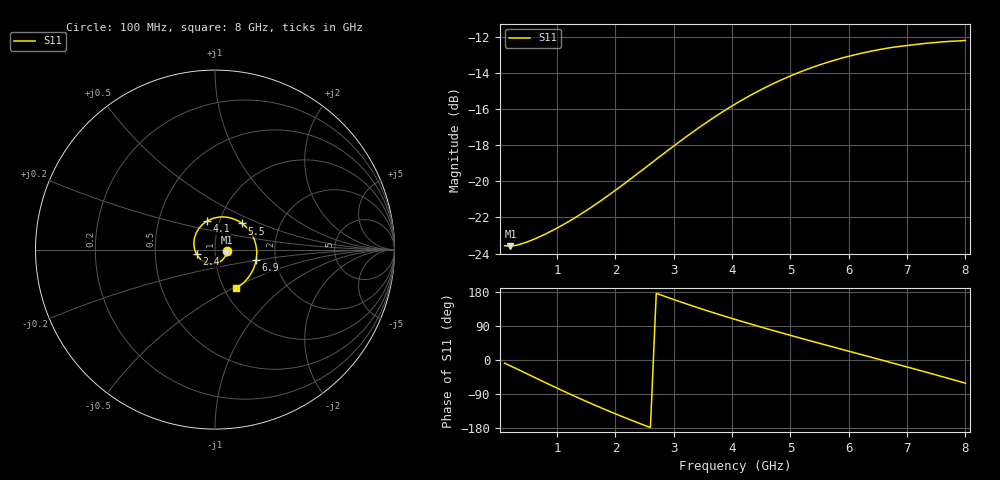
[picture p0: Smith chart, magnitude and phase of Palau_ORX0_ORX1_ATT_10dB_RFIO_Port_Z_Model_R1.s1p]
! Created Fri Oct  9 14:28:06 2020
! Palau ORX0/ORX1 RFIO Port Impedance Model.
! Attenuation  : 10 dB.
! Revision		: R1.
! Impedance Mode 	: Balanced Differential-Mode.
! Impedance Format 	: Series Equivalent Differential Impedance (SEDZ).
# hz S ma R 100
! 1 Port Network Data from SP1.SP block
! freq  magS11  angS11
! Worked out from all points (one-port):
!   80 points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, 100 MHz to 8 GHz, reference 100 ohm
!   lowest |S11| = -23.6 dB at 200 MHz (marker M1), VSWR 1.14, Z = 114 - j4.04 ohm
!   |S11| at or under -10 dB: start of sweep to end of sweep
!   S11 on the Smith chart (normalised r, x): 100 MHz: 1.14, -0.02; 2.4 GHz: 0.81, -0.04; 4.1 GHz: 0.87, +0.29; 5.5 GHz: 1.29, +0.39; 6.9 GHz: 1.58, -0.19; 8 GHz: 1.14, -0.52
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1e8  0.06635 -8.3
2e8  0.06616 -15.5
6e8  0.06911 -45.0
1.1e9  0.07579 -81.4
1.4e9  0.08102 -102.4
1.6e9  0.08504 -116.0
1.8e9  0.08951 -129.2
2.1e9  0.09706 -148.3
2.4e9  0.1056 -166.5
2.8e9  0.1183 170.5
3.1e9  0.1287 154.2
3.3e9  0.1359 143.8
3.6e9  0.1469 128.7
4.1e9  0.1652 104.9
4.4e9  0.1758 91.3
4.6e9  0.1827 82.4
4.9e9  0.1924 69.4
5.1e9  0.1986 60.8
5.5e9  0.2098 44.0
5.8e9  0.2172 31.5
6.1e9  0.2236 19.1
6.5e9  0.2308 2.5
6.7e9  0.2339 -5.8
6.9e9  0.2362 -14.2
7.1e9  0.2384 -22.5
7.5e9  0.2421 -39.5
7.7e9  0.2435 -48.1
8e9  0.2451 -61.2
